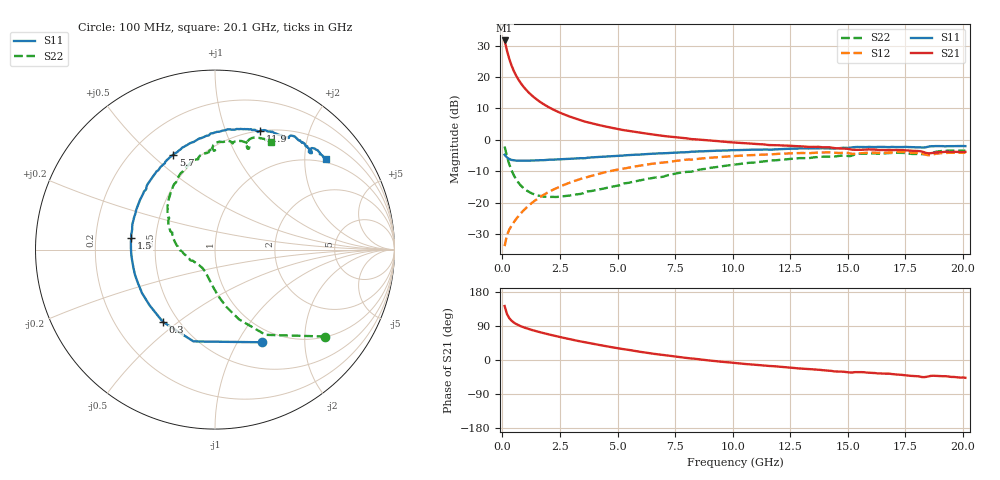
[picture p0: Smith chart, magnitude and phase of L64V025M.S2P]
!  Infineon Technologies AG
! BFR380L3 , PF131585-7, No.6, Th 09.10.01, soldered on pcb-board, measured with PP GSG850
!  Vce=4.0 V,  Ic=25.0 mA
! Common Emitter S-Parameters:  15. November 2001
#  GHz  S  MA  R  50
! f  S11  S21  S12  S22
! GHz  Mag  Ang  Mag  Ang  Mag  Ang  Mag  Ang
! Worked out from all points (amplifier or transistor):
!   201 points, 100 MHz to 20.1 GHz, reference 50 ohm
!   highest |S21| = 31.6 dB at 100 MHz (marker M1)
!   |S21| within 3 dB of that: start of sweep to 195.5 MHz
!   unconditionally stable (mu >= 1): 1.334 GHz to 4.343 GHz
!   at 3.4 GHz: K = 1.02, MAG = 8.5 dB, |S12| = -12.4 dB
!   at 10.1 GHz: K = 0.95, MSG = 2.1 dB, |S12| = -5.2 dB
!   at 20.1 GHz: K = 0.98, MSG = 0.1 dB, |S12| = -4.1 dB
!   S11 on the Smith chart (normalised r, x): 100 MHz: 0.82, -1.27; 300 MHz: 0.41, -0.44; 1.5 GHz: 0.36, +0.06; 5.7 GHz: 0.37, +0.59; 11.9 GHz: 0.50, +1.33; 20.1 GHz: 0.92, +2.51
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0.1  0.5791 -63.1  38.15 142.4  0.02034 65.7  0.7831 -38.2
0.2  0.5254 -103.2  26.56 121.7  0.03023 57.3  0.552 -59.3
0.3  0.4964 -125.9  19.55 110.7  0.03729 55.6  0.4114 -71.0
0.4  0.4788 -139.6  15.28 103.8  0.04301 56.6  0.3269 -78.6
0.5  0.4734 -149.3  12.47 98.8  0.04889 58.4  0.2725 -84.3
0.6  0.468 -156.6  10.52 95.1  0.05504 60.0  0.2353 -88.9
0.7  0.4674 -162.3  9.09 92.0  0.06103 61.3  0.2083 -92.9
0.8  0.4659 -166.8  8.004 89.3  0.06759 62.5  0.1883 -96.4
1  0.4664 -174.4  6.465 84.7  0.08043 64.0  0.1616 -102.7
1.2  0.4682 179.7  5.422 80.8  0.09361 64.6  0.1457 -108.3
1.5  0.4708 172.3  4.379 75.5  0.1135 64.9  0.1316 -116.0
1.8  0.4749 166.3  3.678 70.8  0.1339 64.4  0.1251 -123.0
2.3  0.4859 157.3  2.924 63.5  0.1672 62.6  0.1234 -134.1
2.8  0.4968 149.2  2.443 56.7  0.2002 60.1  0.1286 -143.6
3.5  0.5097 139.2  1.996 47.8  0.2458 56.0  0.1405 -154.0
5.7  0.5784 113.7  1.35 24.3  0.3742 41.7  0.2161 173.0
6.8  0.6084 103.1  1.179 14.5  0.4304 33.9  0.2558 159.0
10.1  0.6845 78.7  0.9055 -8.0  0.5527 12.4  0.4051 127.2
11.9  0.7082 69.1  0.821 -17.0  0.5964 1.7  0.4746 111.5
13.5  0.7307 61.4  0.7736 -24.7  0.6214 -8.3  0.5234 99.9
16.8  0.7667 48.7  0.6905 -36.0  0.6298 -24.3  0.6162 78.6
20.1  0.7948 39.2  0.6426 -46.9  0.6245 -38.1  0.6761 62.3
